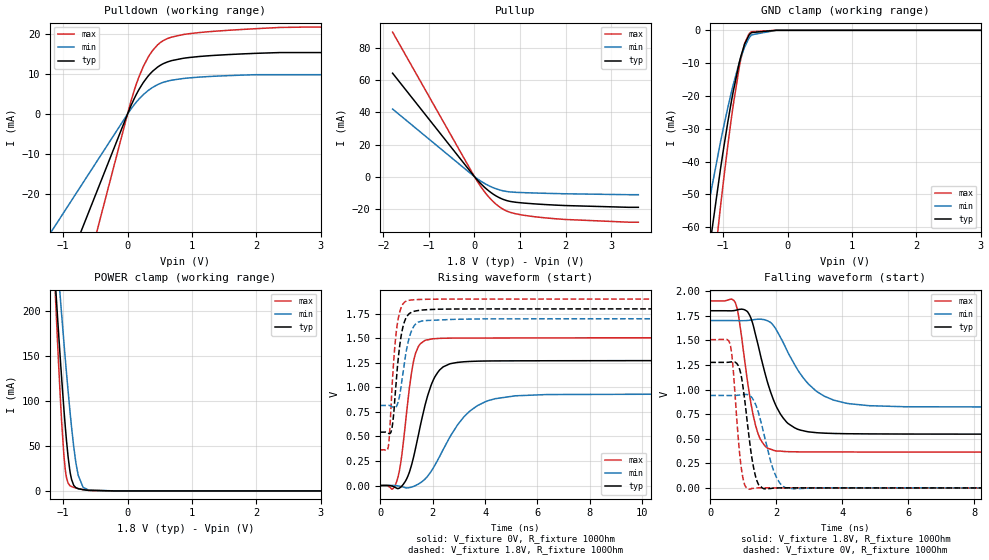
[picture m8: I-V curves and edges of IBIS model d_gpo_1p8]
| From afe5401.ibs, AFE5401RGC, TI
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|   d_gpo_1p8 Model
[Model]   d_gpo_1p8
Model_type   3-state
Polarity   Non-Inverting
Vmeas = 0.9
Vref = 0
Cref = 5pF
Rref = 100
|   typ   min   max
|   (nom PVT)   (fast PVT)   (slow PVT)
C_comp   1.693e-12   1.659e-12   1.738e-12
| Where nom  PVT is Nominal Process, 1.8V, 27C
|   Fast PVT is Strong Process,  1.9V, -40C
|   Slow PVT is Weak Process,   1.7V, 125C
[Voltage Range]   1.8   1.7   1.9
|Junction Temperature
[Temperature Range]   27   125   -40
[Pullup Reference]   1.8   1.7   1.9
[Pulldown Reference]   0   0   0
[Power Clamp Reference]   1.8   1.7   1.9
[GND Clamp Reference]   0   0   0
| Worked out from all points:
|   slope of the pulldown table from 0 to 0.27 V, typ, clamps not added: 31.9 ohm
|   slope of the pullup table from 0 to 0.27 V, typ, clamps not added: 34.6 ohm
|   GND clamp passes 1 mA (typ) near -0.58 V on its own axis
|   POWER clamp passes 1 mA (typ) near -0.65 V on its own axis
|   falling waveform, V_fixture 1.8V, R_fixture 100Ohm: 20-80 % time 675ps typ, 1.04ns min, 423ps max; typ from 1.8 V to 0.544 V
|   rising waveform, V_fixture 0V, R_fixture 100Ohm: 20-80 % time 698ps typ, 1.33ns min, 411ps max; typ from 0 V to 1.27 V
|   rising waveform, V_fixture 1.8V, R_fixture 100Ohm: 20-80 % time 280ps typ, 337ps min, 239ps max; typ from 0.543 V to 1.8 V
|   falling waveform, V_fixture 0V, R_fixture 100Ohm: 20-80 % time 293ps typ, 437ps min, 209ps max; typ from 1.27 V to 0 V
[Pulldown]
|   Voltage   I(typ)   I(min)   I(max)
-1.8V     -73.51mA   -44.92mA   -111.5mA
-84.3mV   -3.443mA   -2.104mA   -5.223mA
39.4mV    1.57mA     944.4uA    2.425mA
111.4mV   4.131mA    2.506mA    6.321mA
238.7mV   7.765mA    4.773mA    11.7mA
392.6mV   10.81mA    6.732mA    16.03mA
474.3mV   11.89mA    7.453mA    17.49mA
567mV     12.75mA    8.037mA    18.57mA
862.2mV   14.01mA    8.935mA    19.97mA
1.546V    14.93mA    9.65mA     21.03mA
2.367V    15.46mA    9.899mA    21.76mA
3.6V      15.46mA    9.899mA    21.85mA
[GND Clamp]
|   Voltage   I(typ)   I(min)   I(max)
-1.8V     -248.3mA   -141.1mA   -369.9mA
-1.355V   -87.44mA   -67.03mA   -111.4mA
-1.264V   -73.66mA   -56.96mA   -94.03mA
-1.251V   -71.69mA   -55.52mA   -91.53mA
-1.042V   -42.28mA   -34.06mA   -53.8mA
-880.4mV  -22.58mA   -19.54mA   -27.97mA
-749.3mV  -9.832mA   -9.781mA   -11.19mA
-665.7mV  -4.149mA   -5.031mA   -4.024mA
-601.5mV  -1.56mA    -2.475mA   -1.184mA
-559.8mV  -686.7uA   -1.383mA   -422uA
-180mV    0A         -265.4nA   0A
3.6V      0A         0A         0A
[Pullup]
|   Voltage   I(typ)   I(min)   I(max)
-1.8V     64.38mA    42.09mA    89.94mA
34.2mV    -1.135mA   -725.1uA   -1.619mA
251.9mV   -7.372mA   -4.679mA   -10.53mA
411.7mV   -10.86mA   -6.845mA   -15.53mA
525.6mV   -12.77mA   -8.005mA   -18.3mA
682mV     -14.62mA   -9.077mA   -21.02mA
795.4mV   -15.43mA   -9.5mA     -22.27mA
1.329V    -16.93mA   -10.15mA   -24.93mA
1.981V    -17.93mA   -10.62mA   -26.59mA
3.6V      -19.04mA   -11.19mA   -28.3mA
[POWER Clamp]
|   Voltage   I(typ)   I(min)   I(max)
-1.8V     1.059A     958.6mA    1.413A
-1.135V   246.4mA    298.1mA    240mA
-1.094V   200.8mA    260.2mA    176.2mA
-1.04V    142.2mA    210.6mA    97.99mA
-986.8mV  89.35mA    163.6mA    38.2mA
-946.9mV  54.97mA    129.9mA    14.38mA
-887.4mV  18.91mA    83.53mA    5.518mA
-834.4mV  6.082mA    48.36mA    3.917mA
-766.4mV  2.485mA    17.42mA    2.633mA
-689.9mV  1.369mA    3.936mA    1.474mA
-601.1mV  588.9uA    933.8uA    530.1uA
3.6V      0A         0A         0A
[Ramp]
R_load = 100
|   typ   min   max
dV/dt_r   0.764329/6.9801e-10   0.560286/1.33011e-09   0.903608/4.09976e-10
dV/dt_f   0.753813/6.72098e-10   0.529083/1.03429e-09   0.922336/4.20725e-10
[Falling Waveform]
V_fixture = 1.8V
V_fixture_min = 1.7V
V_fixture_max = 1.9V
R_fixture = 100Ohm
|   Time   V(typ)   V(min)   V(max)
0s        1.8V       1.7V       1.9V
760ps     1.804V     1.7V       1.881V
1.135ns   1.787V     1.701V     1.065V
1.37ns    1.557V     1.712V     638.2mV
1.625ns   1.208V     1.71V      440.3mV
1.935ns   877.9mV    1.64V      380.8mV
2.355ns   655mV      1.374V     368.6mV
2.98ns    569.8mV    1.054V     366.1mV
4.095ns   551.1mV    862.2mV    365.5mV
14.99ns   543.6mV    818.2mV    362.8mV
[Rising Waveform]
V_fixture = 0V
V_fixture_min = 0V
V_fixture_max = 0V
R_fixture = 100Ohm
|   Time   V(typ)   V(min)   V(max)
0s        1.023nV    76.16nV    424.3pV
640ps     -29.61mV   -2.328mV   51.13mV
815ps     -7.929mV   -11.01mV   296.8mV
1.26ns    277.6mV    -9.924mV   1.253V
1.725ns   834.7mV    70.13mV    1.48V
2.035ns   1.082V     184.4mV    1.496V
2.4ns     1.209V     366.2mV    1.501V
3.225ns   1.262V     708.6mV    1.502V
4.375ns   1.27V      884mV      1.503V
14.99ns   1.274V     933.8mV    1.506V
[Rising Waveform]
V_fixture = 1.8V
V_fixture_min = 1.7V
V_fixture_max = 1.9V
R_fixture = 100Ohm
|   Time   V(typ)   V(min)   V(max)
0s        543.4mV    815.6mV    363.2mV
310ps     532.4mV    816.9mV    398.6mV
435ps     571.5mV    805.7mV    934.4mV
540ps     821.8mV    793.3mV    1.367V
655ps     1.209V     829mV      1.653V
815ps     1.553V     1.048V     1.825V
985ps     1.709V     1.36V      1.879V
1.21ns    1.768V     1.588V     1.891V
1.585ns   1.788V     1.677V     1.897V
14.99ns   1.8V       1.7V       1.9V
[Falling Waveform]
V_fixture = 0V
V_fixture_min = 0V
V_fixture_max = 0V
R_fixture = 100Ohm
|   Time   V(typ)   V(min)   V(max)
0s        1.275V     939.7mV    1.506V
610ps     1.279V     938.7mV    1.449V
935ps     1.143V     946.1mV    214.9mV
1.04ns    901.5mV    949.7mV    34.19mV
1.175ns   518.2mV    941.1mV    -11.67mV
1.325ns   185.5mV    882.9mV    -3.717mV
1.47ns    31mV       752.7mV    1.518mV
1.925ns   -771uV     170.7mV    1.071mV
2.285ns   1.542mV    1.852mV    481.3uV
14.99ns   507.2nV    1.349uV    -24.62nV
